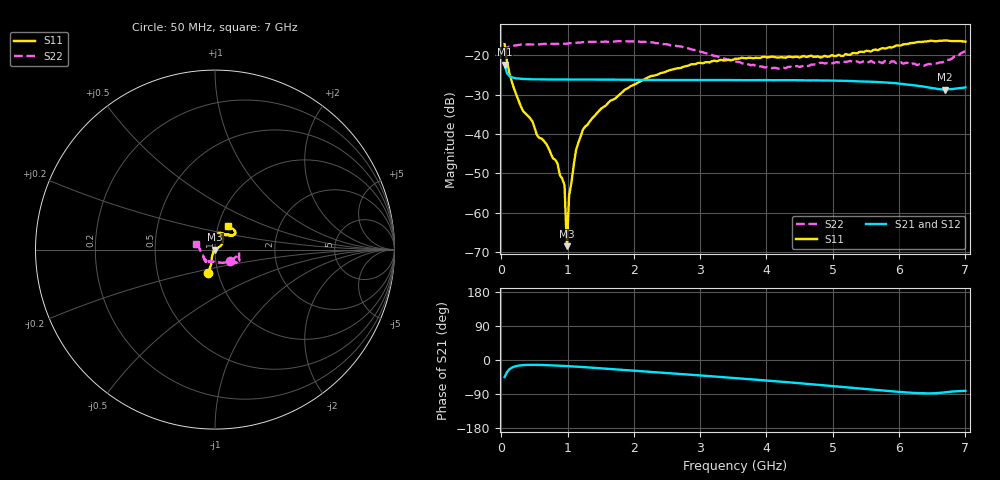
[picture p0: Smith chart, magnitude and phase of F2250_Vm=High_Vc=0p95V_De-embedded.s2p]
! Integrated Device Technology
! Corporate Headquarters
! 6024 Silver Creek Valley Road
! San Jose, CA 95138  USA
! Phone:  1-408-284-8200
! Toll Free:  1-800-223-1366
! Webpage:  http://www.idt.com/
! Timing and RF Division
! 515 Groton Road, Suite 102
! Westford, MA 01886-6024
! Device:  F2250
! Description: Voltage Variable RF Attenuator
! Frequency:  50.0 -  6000.00 MHz
! Package:  3x3 mm Thin QFN Plastic Package: 16 pin
! Ports:  2 RF, 3 DC
!  Pin  1  = GND
!  Pin  2  = NC
!  Pin  3  = RF1  = Port 1
!  Pin  4  = NC
!  Pin  5  = GND
!  Pin  6  = GND
!  Pin  7  = GND
!  Pin  8  = GND
!  Pin  9  = NC
!  Pin 10  = RF2  = Port 2
!  Pin 11  = NC
!  Pin 12  = GND
!  Pin 13  = GND
!  Pin 14  = VCNTRL
!  Pin 15  = VDD
!  Pin 16  = VMODE
! Vcntrl:  0.950 Volts
! Vmode:  +3.300 Volts
! Vdd:  +3.30  Volts
! Current:  1.321 mA
! Data:  The device was measured on a the F2250 evaluation board which has
!  individual transmission lines to the RF pins.  Data was collected
!  using a calibrated network analyzer.  The evaluation board was
!  de-embedded using a TRL calibration technique.
!  The reference plane is the edge of the package pin.
! Misc:  SN 10
!  Action Tracker AT0258
! Date Measured:  2014-11-26
! Date:  2015-10-15  MJV
! Note:
!  Integrated Device Technology supplies this data as a sample of measured
!  data at the package pin for this product.  Your particular data for this
!  product may vary.
!  Data was taken at 25 degrees C.
!  Integrated Device Technology reserves the right to change this data at anytime.
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# GHz S dB R 50
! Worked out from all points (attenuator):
!   201 points, 50 MHz to 7 GHz, reference 50 ohm
!   highest |S21| = -22.35 dB at 50 MHz (marker M1); lowest = -28.7 dB at 6.687 GHz (marker M2)
!   lowest |S11| = -68.5 dB at 988.2 MHz (marker M3), VSWR 1.00, Z = 50 - j0.0371 ohm
!   |S11| at or under -10 dB: start of sweep to end of sweep
!   |S22| runs from -23.4 to -16.4 dB; largest |S21 - S12| = 0.00019
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0.05  -17.20 -106.4  -22.35 -45.0  -22.35 -45.0  -19.50 -37.8
0.1195  -24.36 -108.1  -25.24 -24.9  -25.23 -24.9  -17.84 -12.6
0.29325  -32.94 -118.3  -25.97 -14.1  -25.99 -14.1  -17.29 -9.8
0.467  -36.73 -134.9  -26.11 -12.7  -26.11 -12.7  -17.32 -10.2
0.5365  -40.21 -139.9  -26.10 -12.8  -26.11 -12.8  -17.24 -11.5
0.84925  -47.57 176.0  -26.18 -14.8  -26.18 -14.8  -17.11 -16.9
0.884  -50.47 169.9  -26.20 -15.1  -26.19 -15.1  -17.08 -17.8
0.9535  -52.98 -171.7  -26.17 -15.7  -26.18 -15.7  -17.11 -18.5
0.98825  -68.45 -79.3  -26.18 -16.0  -26.19 -16.0  -17.06 -19.0
1.023  -55.53 15.6  -26.18 -16.3  -26.18 -16.4  -16.97 -19.2
1.12725  -44.04 21.7  -26.19 -17.4  -26.20 -17.4  -16.84 -20.7
1.2315  -38.86 21.9  -26.18 -18.6  -26.18 -18.6  -16.68 -22.5
1.5095  -33.49 30.4  -26.18 -22.0  -26.20 -22.0  -16.60 -25.0
1.857  -28.83 33.2  -26.21 -26.2  -26.22 -26.3  -16.45 -28.0
2.37825  -24.73 42.8  -26.28 -32.7  -26.29 -32.8  -16.92 -31.9
3.525  -20.91 69.9  -26.32 -47.7  -26.32 -47.8  -21.54 -61.1
4.18525  -20.58 76.2  -26.35 -56.6  -26.34 -56.7  -23.44 -97.1
4.7065  -20.37 71.0  -26.37 -64.4  -26.37 -64.4  -22.36 -118.3
5.85325  -17.97 39.6  -27.02 -82.0  -27.00 -82.1  -21.96 -133.3
6.3745  -16.55 40.2  -27.96 -88.1  -27.97 -88.1  -22.66 -152.1
6.68725  -16.26 47.1  -28.74 -85.4  -28.73 -85.5  -21.57 179.2
7  -16.54 61.9  -28.14 -81.3  -28.13 -81.4  -19.00 162.6
